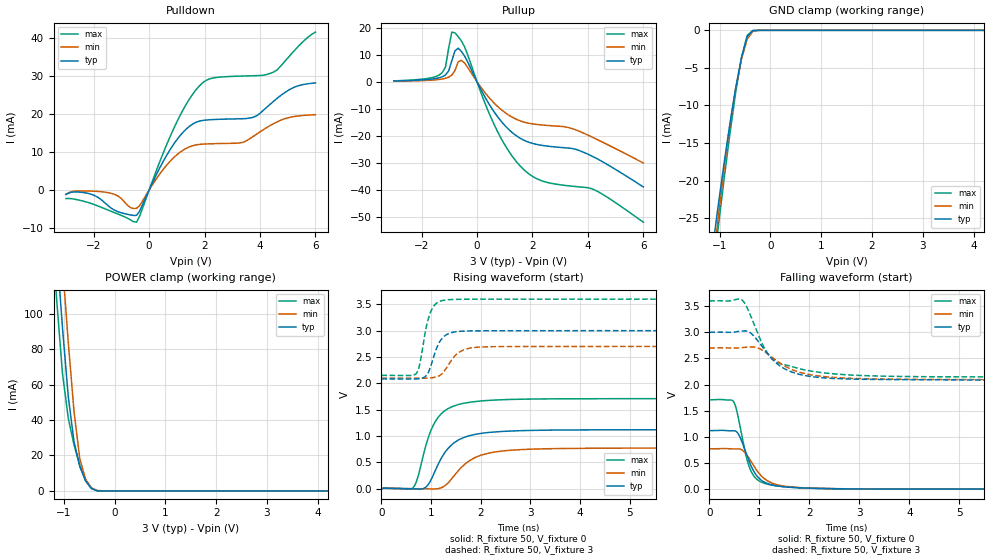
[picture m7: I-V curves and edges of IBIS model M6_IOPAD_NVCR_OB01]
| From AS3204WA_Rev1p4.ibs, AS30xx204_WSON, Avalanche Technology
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[Model] M6_IOPAD_NVCR_OB01
Model_type I/O
Enable   Active-High
Vinl  =  0.9
Vinh  =  2.1
Vmeas =  1.5
Cref  =  30e-12
| Capacitance  typ   min   max
C_comp   3.872127e-12   3.590660e-12   4.176448e-12
| Variables   typ   min   max
[GND Clamp Reference]   0   0   0
[POWER Clamp Reference]   3   2.7   3.6
[Pulldown Reference]   0   0   0
[Pullup Reference]   3   2.7   3.6
[Temperature Range]   25   105   -40
[Voltage Range]   3   2.7   3.6
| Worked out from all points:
|   slope of the pulldown table from 0 to 0.45 V, typ, clamps not added: 66.9 ohm
|   slope of the pullup table from 0 to 0.45 V, typ, clamps not added: 53.1 ohm
|   GND clamp passes 1 mA (typ) near -0.46 V on its own axis
|   POWER clamp passes 1 mA (typ) near -0.42 V on its own axis
|   falling waveform, R_fixture 50, V_fixture 0: 20-80 % time 321ps typ, 395ps min, 255ps max; typ from 1.12 V to 0 V
|   falling waveform, R_fixture 50, V_fixture 3: 20-80 % time 599ps typ, 707ps min, 504ps max; typ from 3 V to 2.08 V
|   rising waveform, R_fixture 50, V_fixture 0: 20-80 % time 475ps typ, 569ps min, 386ps max; typ from 0 V to 1.12 V
|   rising waveform, R_fixture 50, V_fixture 3: 20-80 % time 221ps typ, 296ps min, 185ps max; typ from 2.08 V to 3 V
[GND Clamp]
| Voltage   I(typ)   I(min)   I(max)
-3V       -145.9mA   -151.9mA   -144.2mA
-1.138V   -29.07mA   -31.55mA   -32.68mA
-1.024V   -23.24mA   -24.83mA   -26.15mA
-910.3mV  -17.69mA   -18.46mA   -19.83mA
-796.6mV  -12.47mA   -12.67mA   -13.82mA
-682.8mV  -7.718mA   -7.754mA   -8.316mA
-569mV    -3.663mA   -3.867mA   -3.675mA
-455.2mV  -839.2uA   -1.152mA   -666.1uA
-341.4mV  -35.63uA   -111.1uA   -11.17uA
-113.8mV  -8.642nA   -188.3nA   -1.888nA
6V        0A         0A         0A
[POWER Clamp]
| Voltage   I(typ)   I(min)   I(max)
-3V       949.8mA    984.2mA    923.5mA
-1.252V   183.6mA    221.4mA    154mA
-1.138V   136.7mA    174.2mA    107.6mA
-1.024V   92.09mA    128.1mA    66.35mA
-910.3mV  53.33mA    83.97mA    41.06mA
-796.6mV  27.72mA    44.75mA    25.94mA
-682.8mV  13.75mA    18.06mA    14.29mA
-569mV    5.664mA    6.605mA    5.738mA
-455.2mV  1.446mA    1.789mA    1.305mA
-341.4mV  77.09uA    287.6uA    62.73uA
-227.6mV  1.148uA    12.92uA    332nA
6V        0A         0A         0A
[Pulldown]
| Voltage   I(typ)   I(min)   I(max)
-3V       -1.178mA   -1.11mA    -2.252mA
-2.162V   -950.8uA   -265.9uA   -3.362mA
-1.479V   -4.121mA   -692.7uA   -5.266mA
-455.2mV  -6.659mA   -4.795mA   -8.439mA
827.6mV   11.41mA    8.082mA    15.18mA
1.759V    17.96mA    11.91mA    26.89mA
2.276V    18.48mA    12.15mA    29.35mA
3.372V    18.7mA     12.49mA    29.9mA
3.745V    19.07mA    14.02mA    29.98mA
4.49V     23.28mA    17.41mA    30.94mA
5.234V    26.97mA    19.29mA    36.55mA
6V        28.1mA     19.77mA    41.44mA
[Pullup]
| Voltage   I(typ)   I(min)   I(max)
-3V       306.9uA    228.8uA    360.3uA
-1.366V   1.498mA    877.1uA    2.527mA
-1.138V   2.564mA    1.314mA    5.499mA
-1.024V   4.04mA     1.741mA    12.49mA
-910.3mV  7.819mA    2.481mA    18.38mA
-796.6mV  11.48mA    4.213mA    18.09mA
-569mV    11.29mA    7.95mA     15.19mA
620.7mV   -11.18mA   -7.898mA   -15.89mA
1.655V    -21.41mA   -14.76mA   -32.13mA
2.379V    -23.53mA   -15.98mA   -36.72mA
3.745V    -25.61mA   -18.52mA   -38.87mA
6V        -38.84mA   -29.98mA   -51.86mA
[Ramp]
dV/dt_r   0.671391/0.474616n  0.462683/0.568662n  1.02545/0.385509n
dV/dt_f   0.55145/0.59859n  0.363091/0.707295n  0.872156/0.50432n
R_load = 50
[Falling Waveform]
R_fixture = 50
V_fixture = 0
V_fixture_min = 0
V_fixture_max = 0
| Time   V(typ)   V(min)   V(max)
0s        1.119V     771.1mV    1.709V
473.4ps   1.118V     770.5mV    1.686V
533.2ps   1.106V     771.1mV    1.555V
593.2ps   1.034V     770.2mV    1.298V
728.9ps   703.6mV    678.2mV    653.8mV
863.5ps   386.6mV    483.4mV    288.7mV
1.016ns   188.4mV    277.1mV    146.3mV
1.166ns   106.1mV    156.6mV    93.77mV
1.528ns   42.92mV    52.9mV     43.77mV
21.88ns   384.8nV    503.1nV    8.699uV
[Falling Waveform]
R_fixture = 50
V_fixture = 3
V_fixture_min = 2.7
V_fixture_max = 3.6
| Time   V(typ)   V(min)   V(max)
0s        3V         2.7V       3.6V
657.7ps   3.026V     2.71V      3.615V
831.8ps   2.984V     2.721V     3.301V
1.084ns   2.691V     2.643V     2.73V
1.186ns   2.563V     2.573V     2.57V
1.324ns   2.424V     2.471V     2.441V
1.551ns   2.279V     2.331V     2.372V
1.808ns   2.194V     2.235V     2.302V
2.743ns   2.107V     2.124V     2.187V
21.88ns   2.081V     2.095V     2.146V
[Rising Waveform]
R_fixture = 50
V_fixture = 0
V_fixture_min = 0
V_fixture_max = 0
| Time   V(typ)   V(min)   V(max)
0s        324.6nV    434.9nV    8.69uV
624.3ps   -2.1mV     963.2uV    7.487mV
734.1ps   -6.735mV   -177.1uV   219.7mV
907.3ps   39.49mV    -3.379mV   860.6mV
1.128ns   434.2mV    -1.573mV   1.337V
1.475ns   879mV      258.4mV    1.575V
1.751ns   1V         516.1mV    1.637V
2.01ns    1.051V     637.2mV    1.666V
4.026ns   1.116V     766.2mV    1.708V
21.88ns   1.119V     771.1mV    1.709V
[Rising Waveform]
R_fixture = 50
V_fixture = 3
V_fixture_min = 2.7
V_fixture_max = 3.6
| Time   V(typ)   V(min)   V(max)
0s        2.081V     2.095V     2.146V
705ps     2.083V     2.096V     2.19V
773.5ps   2.089V     2.096V     2.37V
887.1ps   2.13V      2.097V     2.998V
1.012ns   2.382V     2.105V     3.402V
1.161ns   2.769V     2.142V     3.551V
1.364ns   2.948V     2.373V     3.59V
1.655ns   2.992V     2.635V     3.597V
2.161ns   2.998V     2.695V     3.599V
21.88ns   3V         2.7V       3.6V
